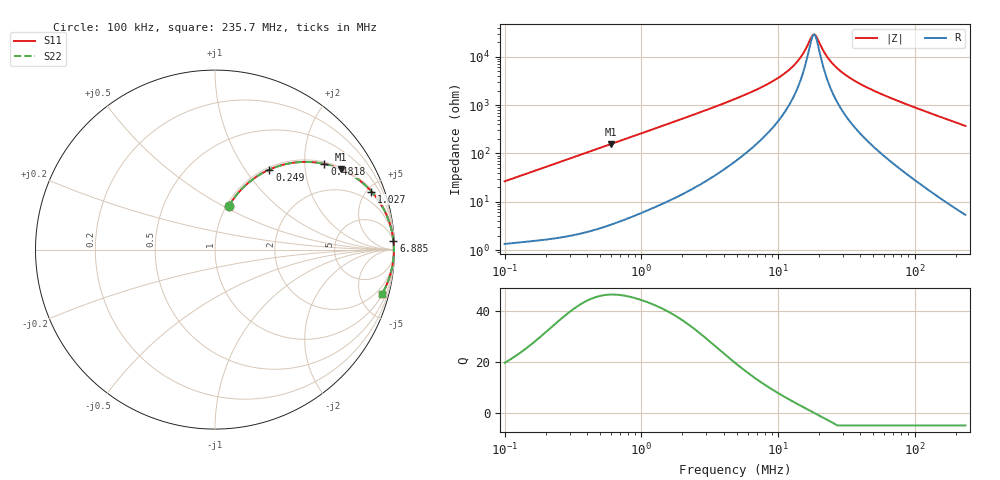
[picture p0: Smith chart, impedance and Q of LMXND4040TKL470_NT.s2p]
! LMXND4040TKL470_NT  S-PARAMETER MODEL  ( Standard Model )
! Model Generated by TAIYO YUDEN Corporation (https://www.yuden.co.jp/en/)
! Version 1.0
! TAIYO YUDEN Control No. 20250409
! Copyright(c) 2025 TAIYO YUDEN CO.,LTD. All Rights Reserved.
! Product Description (link to TY-COMPAS)
! https://ds.yuden.co.jp/TYCOMPAS/or/detail?pn=LMXND4040TKL470MNT&u=M
! Products Name : Inductors
! Characteristics :
!  Inductance : 47 [uH] , SRF(min) : 10 [MHz] , DC Resistance(max) : 0.78 [Ohm]
!  Rated Current : Saturation  600 [mA] , Temp Rise  730 [mA] (40 [degC])
!  Case Size : 4.0 x 4.0 / 0.157 x 0.157 [mm/inch] , Thickness : 1.8 / 0.071 [mm/inch]
!  (Conditions: Temperature = 25 [degC] , DC Bias Current = 0 [A])
! External Node Assignments :
!  1  o---GGG---o  2
! GND o---------o GND
! Frequency Range : 0.1MHz  -  235.669543MHz  [ 402 STEP ]
# MHz S RI R 50
! Freq[MHz].  S11 Real  S11 Imag  S21 Real  S21 Imag  S12 Real  S12 Imag  S22 Real  S22 Imag
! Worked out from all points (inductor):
!   401 points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, 100 kHz to 235.7 MHz, reference 50 ohm
!   read as one part in series: L = 41.9 uH near 104 kHz
!   highest Q = 46.6 at 596.5 kHz (marker M1), where L = 41.4 uH
!   self-resonance near 18.17 MHz
!   S11 on the Smith chart (normalised r, x): 100 kHz: 1.03, +0.53; 249 kHz: 1.04, +1.30; 481.8 kHz: 1.05, +2.51; 1.027 MHz: 1.12, +5.34; 6.885 MHz: 4, +41; 235.7 MHz: 1.11, -7.42
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0.1  0.0761 0.241  0.9239 -0.241  0.9239 -0.241  0.0761 0.241
0.159345  0.158 0.3469  0.842 -0.3469  0.842 -0.3469  0.158 0.3469
0.249027  0.303 0.446  0.697 -0.446  0.697 -0.446  0.303 0.446
0.367165  0.4793 0.4881  0.5207 -0.4881  0.5207 -0.4881  0.4793 0.4881
0.481827  0.6098 0.477  0.3902 -0.477  0.3902 -0.477  0.6098 0.477
0.596527  0.7032 0.4463  0.2968 -0.4463  0.2968 -0.4463  0.7032 0.4463
1.027285  0.8715 0.3236  0.1285 -0.3236  0.1285 -0.3236  0.8715 0.3236
1.348099  0.9194 0.2605  0.0806 -0.2605  0.0806 -0.2605  0.9194 0.2605
2.460794  0.9722 0.1499  0.0278 -0.1499  0.0278 -0.1499  0.9722 0.1499
4.854581  0.9908 0.0736  0.00922 -0.0736  0.00922 -0.0736  0.9908 0.0736
6.885023  0.9941 0.0481  0.00591 -0.0481  0.00591 -0.0481  0.9941 0.0481
9.764703  0.9957 0.0284  0.0043 -0.0284  0.0043 -0.0284  0.9957 0.0284
12.56779  0.9963 0.0164  0.00373 -0.0164  0.00373 -0.0164  0.9963 0.0164
14.96703  0.9965 0.00872  0.00352 -0.00872  0.00352 -0.00872  0.9965 0.00872
17.8243  0.9966 0.00131  0.00343 -0.00131  0.00343 -0.00131  0.9966 0.00131
18.89317  0.9966 -0.00113  0.00343 0.00113  0.00343 0.00113  0.9966 -0.00113
23.3907  0.9965 -0.0102  0.00353 0.0102  0.00353 0.0102  0.9965 -0.0102
29.52652  0.9962 -0.0206  0.00385 0.0206  0.00385 0.0206  0.9962 -0.0206
41.07099  0.9952 -0.0375  0.00483 0.0375  0.00483 0.0375  0.9952 -0.0375
65.44454  0.9918 -0.0686  0.00818 0.0686  0.00818 0.0686  0.9918 -0.0686
126.6249  0.9767 -0.1388  0.0233 0.1388  0.0233 0.1388  0.9767 -0.1388
235.6695  0.9292 -0.2495  0.0708 0.2495  0.0708 0.2495  0.9292 -0.2495
